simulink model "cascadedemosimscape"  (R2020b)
settings: Solver=ode4  StartTime=0.0  StopTime=0.025  FixedStep=0.0001  RelTol=1e-3  AbsTol=1e-3
libraries: fl_lib x7, nesl_utility x3

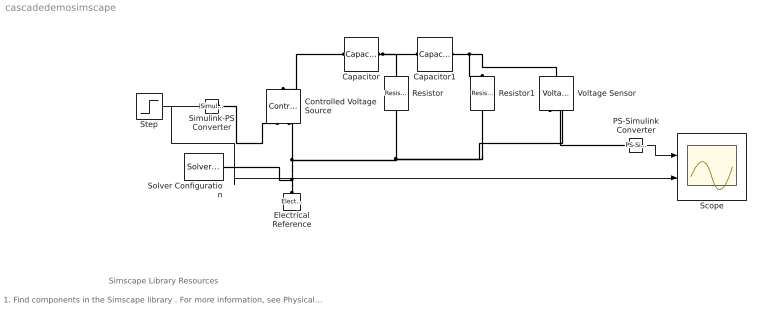
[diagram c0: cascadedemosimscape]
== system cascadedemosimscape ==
  note: 1. Find components in the Simscape library . For more information, see Physical Modeling - Blocks . 2. Connect the components to form a physical network. For more information, see Essential Steps for Constructing a Physical Model . 3. Explore simulation results using sscexplore
  note: Simscape Library Resources
  Capacitor : fl_lib/Electrical/Electrical Elements/Capacitor  c=1 uF  r=1e-6 Ohm  g=0 1/Ohm  i_specify=off  i_priority=None  i=0 A  i_nominal_specify=off  i_nominal_unit=A  i_nominal_value=1  v_specify=off  v_priority=None  v=0 V  v_nominal_specify=off  v_nominal_unit=V  v_nominal_value=1  vc_specify=off  vc_priority=High  vc=0 V  vc_nominal_specify=off  vc_nominal_unit=V  vc_nominal_value=1
  Capacitor1 : fl_lib/Electrical/Electrical Elements/Capacitor  c=1 uF  r=1e-6 Ohm  g=0 1/Ohm  i_specify=off  i_priority=None  i=0 A  i_nominal_specify=off  i_nominal_unit=A  i_nominal_value=1  v_specify=off  v_priority=None  v=0 V  v_nominal_specify=off  v_nominal_unit=V  v_nominal_value=1  vc_specify=off  vc_priority=High  vc=0 V  vc_nominal_specify=off  vc_nominal_unit=V  vc_nominal_value=1
  Controlled Voltage Source : fl_lib/Electrical/Electrical Sources/Controlled Voltage Source
  Electrical Reference : fl_lib/Electrical/Electrical Elements/Electrical Reference
  PS-Simulink Converter : nesl_utility/PS-Simulink Converter  PhysicalDomain=network_engine_domain  SubClassName=ps_output  LeftPortType=input  RightPortType=output  PseudoPeriodic=off  Frequencies=[]  Unit=inherit  AffineConversion=off
  Resistor : fl_lib/Electrical/Electrical Elements/Resistor  R=1 kOhm  i_specify=off  i_priority=None  i=0 A  i_nominal_specify=off  i_nominal_unit=A  i_nominal_value=1  v_specify=off  v_priority=None  v=0 V  v_nominal_specify=off  v_nominal_unit=V  v_nominal_value=1
  Resistor1 : fl_lib/Electrical/Electrical Elements/Resistor  R=1 kOhm  i_specify=off  i_priority=None  i=0 A  i_nominal_specify=off  i_nominal_unit=A  i_nominal_value=1  v_specify=off  v_priority=None  v=0 V  v_nominal_specify=off  v_nominal_unit=V  v_nominal_value=1
  Scope : Scope  NumInputPorts=2
  Simulink-PS Converter : nesl_utility/Simulink-PS Converter  PhysicalDomain=network_engine_domain  SubClassName=ps_input  LeftPortType=input  RightPortType=output  PseudoPeriodic=off  Frequencies=[]  NoiseDistribution=none  NoiseParameters=[]  Unit=1  AffineConversion=off  FilteringAndDerivatives=provide  SimscapeFilterOrder=1  InputFilterTimeConstant=0.001  UdotUserProvided=0
  Solver Configuration : nesl_utility/Solver Configuration  PhysicalDomain=network_engine_domain  SubClassName=solver  LeftPortType=input  RightPortType=generic  Tones=[]  Harmonics=[]  SimulateNoise=off  Profile=off  UseLocalSampling=off  EnableSwitchedLinearOptims=on  FrequencyDomain=off  UseCCode=off  RelTol=0.001  AbsTol=1e-06  MinStep=1e-09  ToWorkspace=off  RevertToSquareIcSolve=off  NumHomotopyIterations=100  PhasorMode=off  PhasorModeNumHarmonics=1  DoDC=off  ResidualTolerance=1e-09  UseLocalSolver=off  LocalSolverChoice=NE_BACKWARD_EULER_ADVANCER  LocalSolverSampleTime=0.001  DoFixedCost=off  MaxNonlinIter=3  MaxModeIter=2  ComputeImpulses=off  ImpulseIterations=2  LinearAlgebra=auto  EquationFormulation=NE_TIME_EF  DelaysMemoryBudget=1024  AutomaticFiltering=on  FilteringTimeConstant=0.001  PartitionStorageMethod=AS_NEEDED  PartitionMemoryBudget=1024  PartitionMethod=ROBUST
  Step : Step  Time=0.001  SampleTime=0
  Voltage Sensor : fl_lib/Electrical/Electrical Sensors/Voltage Sensor
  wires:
  PS-Simulink Converter/1 -> Scope/1
  Step/1 -> Scope/2, Simulink-PS Converter/1
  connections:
  Simulink-PS Converter/RConn1 -- Controlled Voltage Source/RConn1
  Electrical Reference/LConn1 -- Solver Configuration/RConn1 -- Voltage Sensor/RConn2 -- Resistor1/RConn1 -- Resistor/RConn1 -- Controlled Voltage Source/RConn2
  Capacitor/RConn1 -- Controlled Voltage Source/LConn1
  Capacitor/LConn1 -- Resistor/LConn1 -- Capacitor1/RConn1
  Capacitor1/LConn1 -- Voltage Sensor/LConn1 -- Resistor1/LConn1
  PS-Simulink Converter/LConn1 -- Voltage Sensor/RConn1
